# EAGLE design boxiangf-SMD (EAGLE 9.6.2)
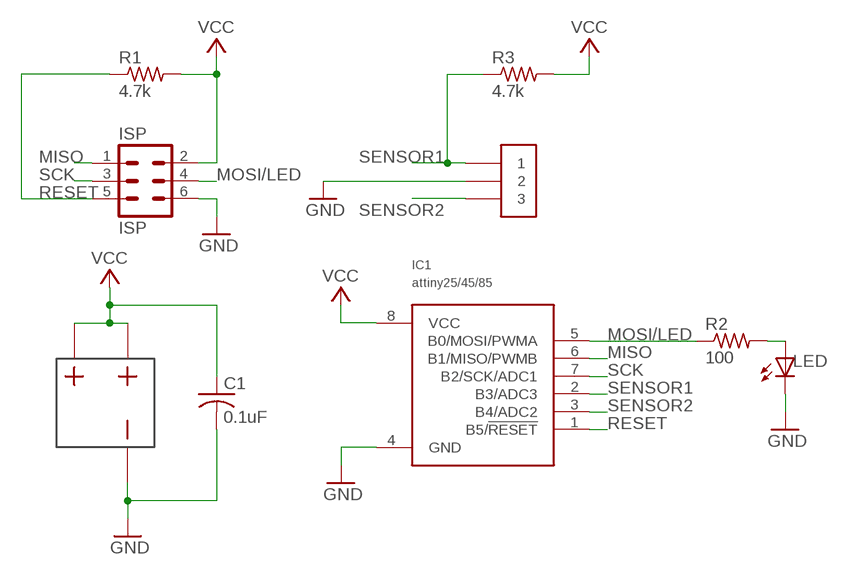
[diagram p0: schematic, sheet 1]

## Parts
C1  0.1uF  CAPACITORSM_CAP  [C0402]
IC1  attiny25/45/85  ATTINY25SM_ATTINY  [8S1]
ISP  ISP  6PINCON_ISPSM_6PIN  [SM6PIN]
LED  LEDSMLED  [CHIPLED_0603]
R1  4.7k  RESISTORSMRESISTOR  [R0402]
R2  100  RESISTORSMRESISTOR  [R0402]
R3  4.7k  RESISTORSMRESISTOR  [R0402]
SENSE  3PINCONSM_3PIN  [SM3PIN]
US1  BATTERYSM_BA2032  [BA2032SM]

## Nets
GND: C1.2 IC1.4(GND) ISP.6 LED.C SENSE.2 US1.1
MISO: IC1.6(B1/MISO/PWMB) ISP.1
MOSI/LED: IC1.5(B0/MOSI/PWMA) ISP.4 R2.1
N$2: LED.A R2.2
RESET: IC1.1(B5/!RESET) ISP.5 R1.1
SCK: IC1.7(B2/SCK/ADC1) ISP.3
SENSOR1: IC1.2(B3/ADC3) R3.1 SENSE.1
SENSOR2: IC1.3(B4/ADC2) SENSE.3
VCC: C1.1 IC1.8(VCC) ISP.2 R1.2 R3.2 US1.2 US1.3

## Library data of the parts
C1 = TinyGadget:CAPACITOR
IC1 = TinyGadget:ATTINY25
ISP = TinyGadget:6PINCON_ISP
LED = TinyGadget:LED
R1-R3 = TinyGadget:RESISTOR
SENSE = TinyGadget:3PINCON
US1 = TinyGadget:BATTERY

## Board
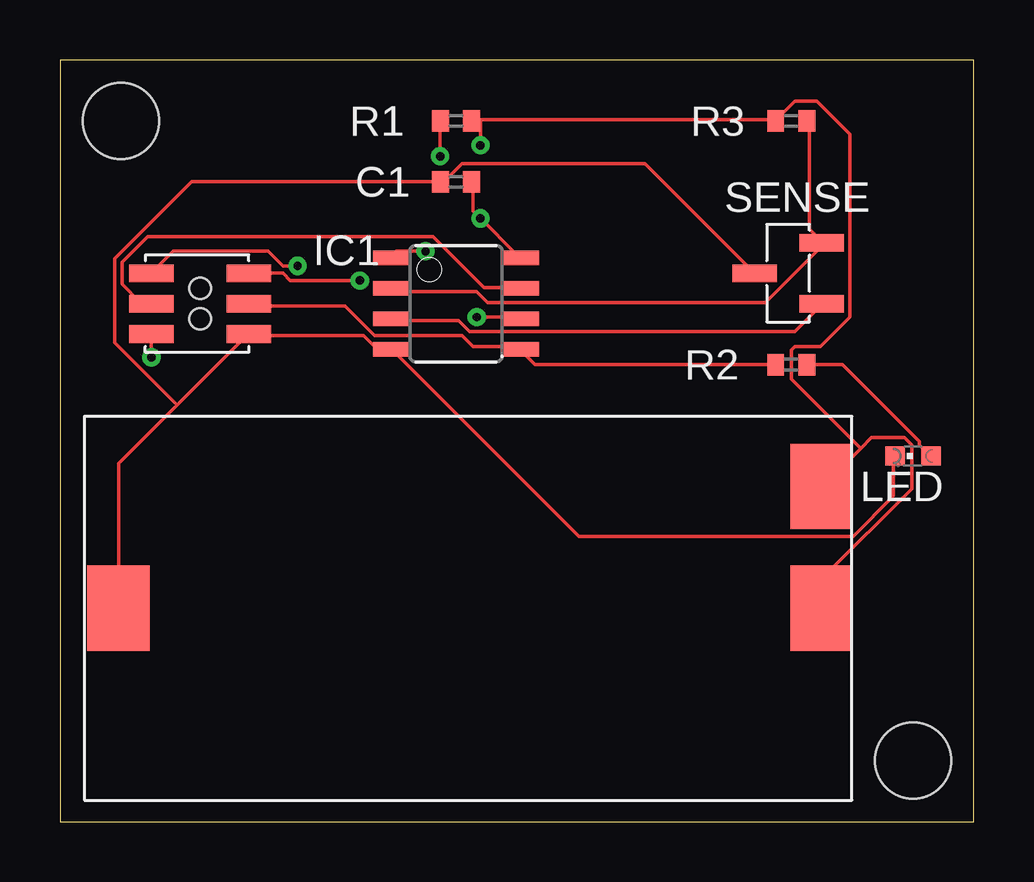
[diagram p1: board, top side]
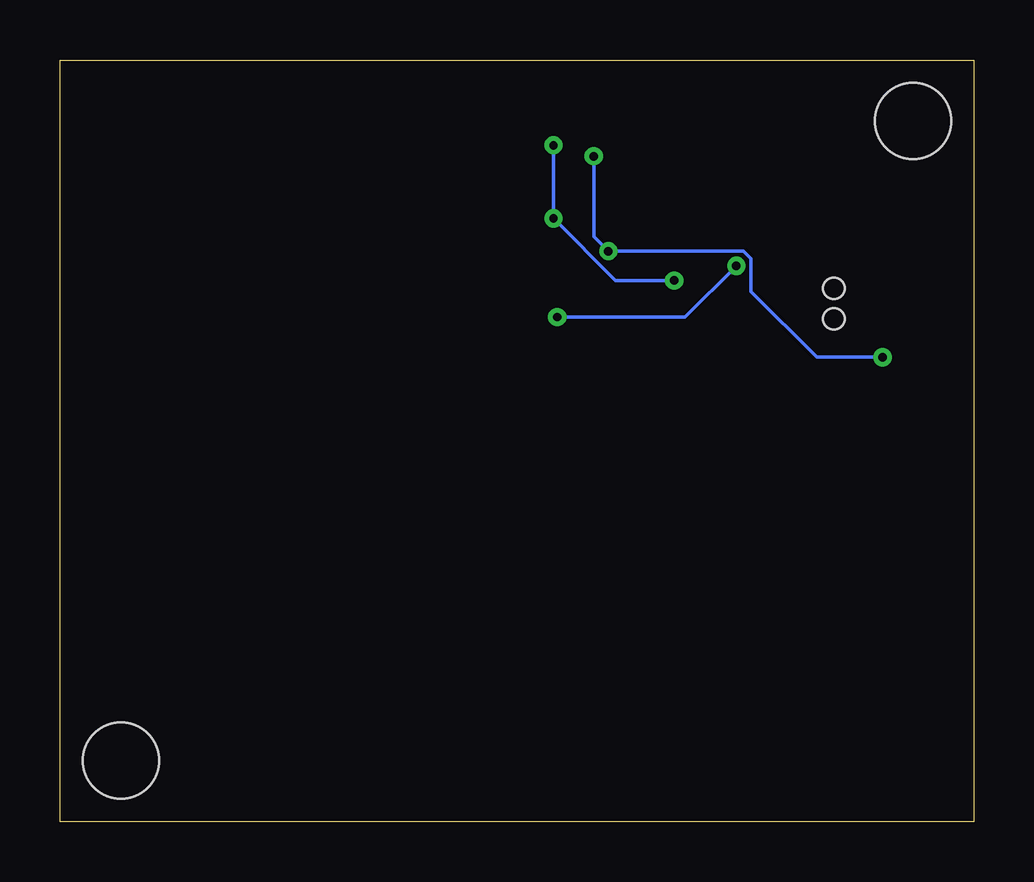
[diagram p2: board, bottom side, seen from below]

Size 38.1 x 31.75 mm. Coordinates in mm from the lower left corner, seen from the top.
Outline: 0,0 38.1,0 38.1,31.75 0,31.75 0,0
Copper layers (1*16): Top 0.035mm / dielectric 1.5mm / Bottom 0.035mm
Design rules "default *": minimum track width 6mil, minimum drill 0.35mm, track to track 6mil, track to pad 6mil, pad to pad 6mil, via to via 6mil, smd to smd 6mil, copper to edge 25mil, drill to drill 6mil, minimum pad ring 10mil, minimum via ring 8mil, stop-mask expansion 4mil, vias tented up to drill 0mil, thermal gap 5mil
Holes 3.17 mm at 2.54,29.21 35.56,2.54

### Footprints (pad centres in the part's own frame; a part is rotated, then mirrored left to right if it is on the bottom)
C0402 = smd 0.7 x 0.9: 1 -0.65,0; 2 0.65,0
8S1 = smd 0.6 x 1.6: 1 -1.905,-2.654; 2 -0.645,-2.654; 3 0.625,-2.654; 4 1.895,-2.654; 5 1.905,2.654; 6 0.635,2.654; 7 -0.635,2.654; 8 -1.905,2.654
SM6PIN = smd 0.737 x 1.854: 1 0,-1.27; 2 0,2.794; 3 1.27,-1.27; 4 1.27,2.794; 5 2.54,-1.27; 6 2.54,2.794 | hole 0.889: 0.635,0.762; 1.905,0.762
CHIPLED_0603 = smd 0.8 x 0.8: A 0,-0.75; C 0,0.75
R0402 = smd 0.7 x 0.9: 1 -0.65,0; 2 0.65,0
SM3PIN = smd 0.737 x 1.854: 1 0,0; 2 1.27,-2.794; 3 2.54,0
BA2032SM = smd 2.591 x 3.556: 1 29.312,0; 2 0,-5.08; 3 0,0

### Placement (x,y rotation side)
C1  16.51,26.67 180 top
IC1  16.51,21.59 270 top
ISP  5.08,22.86 270 top
LED  35.56,15.24 90 top
R1  16.51,29.21 0 top
R2  30.48,19.05 0 top
R3  30.48,29.21 180 top
SENSE  31.75,24.13 270 top
US1  31.75,8.89 180 top

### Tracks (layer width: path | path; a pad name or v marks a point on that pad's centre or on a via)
GND
  Top 0.152: SENSE.2 24.38,27.43 16.76,27.43 16,26.67 C1.2 5.49,26.67 2.29,23.47 2.29,19.96 4.88,17.37 | LED.C 34.75,15.24 34.75,13.56 33.07,11.89 21.64,11.89 13.87,19.66 IC1.4 13.72,19.81 13.11,19.81 12.65,20.27 7.92,20.27 ISP.6 7.77,20.27 4.88,17.37 | US1.1 2.44,14.94 4.88,17.37
MISO  (via drill 0.35)
  Top 0.152: v17.37,21.03 19.05,21.03 IC1.6 | v9.91,23.16 9.3,23.16 8.69,23.77 4.72,23.77 ISP.1
  Bottom 0.152: v17.37,21.03 12.04,21.03 v9.91,23.16
MOSI/LED
  Top 0.152: R2.1 19.81,19.05 19.2,19.66 IC1.5 19.05,19.81 17.22,19.81 16.76,20.27 13.11,20.27 11.89,21.49 7.92,21.49 ISP.4
N$2
  Top 0.152: R2.2 32.61,19.05 35.81,15.85 35.81,15.7 36.27,15.24 LED.A
RESET  (via drill 0.35)
  Top 0.152: v15.85,27.74 15.85,29.11 R1.1 | v15.24,23.77 14.02,23.77 13.87,23.62 IC1.1 | v3.81,19.36 ISP.5
  Bottom 0.152: v15.85,27.74 15.85,24.38 v15.24,23.77 9.6,23.77 9.3,23.47 9.3,22.1 6.55,19.36 v3.81,19.36
SCK
  Top 0.152: IC1.7 19.05,22.25 17.68,22.25 15.54,24.38 3.66,24.38 2.59,23.32 2.59,22.4 3.35,21.64 3.81,21.64 ISP.3
SENSOR1
  Top 0.152: R3.1 31.24,29.11 31.24,24.69 31.7,24.23 SENSE.1 31.85,24.08 29.41,21.64 17.83,21.64 17.37,22.1 13.87,22.1 IC1.2
SENSOR2
  Top 0.152: IC1.3 13.87,20.88 16.61,20.88 17.07,20.42 30.63,20.42 31.7,21.49 SENSE.3
VCC  (via drill 0.35)
  Top 0.152: C1.1 17.22,26.67 17.22,25.45 v17.53,25.15 19.05,23.62 IC1.8 | ISP.2 9.3,22.86 9.6,22.55 v12.5,22.55 | 17.53,29.26 29.72,29.26 R3.2 29.87,29.26 30.63,30.02 31.55,30.02 32.92,28.65 32.92,21.03 31.7,19.81 30.63,19.81 30.48,19.66 30.48,18.44 33.38,15.54 | 17.53,29.26 17.22,29.26 R1.2 | 33.38,15.54 31.85,14.02 US1.2 | 33.38,15.54 33.83,16 35.2,16 35.51,15.7 35.51,13.87 31.85,10.21 31.85,8.99 US1.3 | 17.53,29.26 v17.53,28.19
  Bottom 0.152: v12.5,22.55 14.94,22.55 v17.53,25.15 v17.53,28.19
